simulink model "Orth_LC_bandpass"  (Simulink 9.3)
settings: Solver=VariableStepAuto  StartTime=0.0  StopTime=1  RelTol=1e-3
InitFcn:
  | Test_LibVishia_Ctrl.TestOrthOsc_init();
  | TstepHw=0.000001;
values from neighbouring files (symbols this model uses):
  Tstep = 0.000050    (= 5e-05)    [TestOrthOsc_init.m]    (also in Test_PIDctrl_init.m = 0.0001)
libraries: powerlib x12, libVishia_Ctrl x4, libVishia_Conv x2, libVishia_CtrlSfn x1, simulink x1

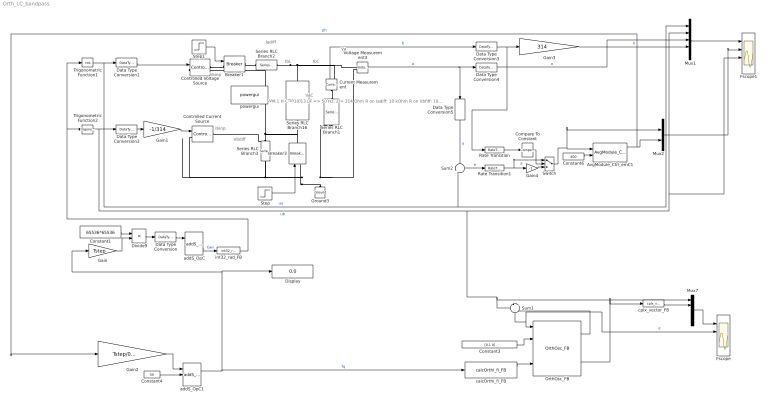
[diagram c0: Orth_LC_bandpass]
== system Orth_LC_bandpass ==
  note: L = 1 H C = 10.13 µF => 50 Hz, Z = 314 Ohm R on Iadiff: 10 kOhm R on Vbfiff: 10 Ohm => k ~ 0.03
  note: VaC
  note: Vainp
  note: Ibinp
  note: Vbdiff
  note: Iadiff
  note: IbC
  note: Va
  note: IbL
  note: VaL
  AvgModule_Ctrl_emC1 : libVishia_CtrlSfn/AvgModule_Ctrl_emC  SystemSampleTime=-1
  Breaker1 : powerlib/Elements/Breaker  InitialState=0  SwitchingTimes="[1/60  5/60]"  External=on  BreakerResistance=0.01  SnubberResistance=1e6  SnubberCapacitance=inf  Measurements=None  MoreParameters=on  NoBreakLoop=off
  Breaker3 : powerlib/Elements/Breaker  InitialState=0  SwitchingTimes="[1/60  5/60]"  External=on  BreakerResistance=0.01  SnubberResistance=1e6  SnubberCapacitance=inf  Measurements=None  MoreParameters=on  NoBreakLoop=off
  Compare To Constant : simulink/Logic and Bit Operations/Compare To Constant  relop=>=  const=0  OutDataTypeStr=boolean
  Constant1 : Constant  Value=65536*65536  OutDataTypeStr=single
  Constant3 : Constant  Value=[0.1 0]  OutDataTypeStr=single
  Constant4 : Constant  Value=50  OutDataTypeStr=single
  Constant6 : Constant  Value=400  OutDataTypeStr=single
  Controlled Current Source : powerlib/Electrical Sources/Controlled Current Source  Initialize=on  Source_Type=AC  Amplitude=0  Phase=0  Frequency=0  Measurements=None
  Controlled Voltage Source : powerlib/Electrical Sources/Controlled Voltage Source  Initialize=on  Source_Type=AC  Amplitude=0  Phase=0  Frequency=0  Measurements=None
  Current Measurement : powerlib/Measurements/Current Measurement  PhasorSimulation=off  OutputType=Complex  PSBequivalent=0
  Data Type Conversion : DataTypeConversion  OutDataTypeStr=int32
  Data Type Conversion1 : DataTypeConversion  OutDataTypeStr=double
  Data Type Conversion2 : DataTypeConversion  OutDataTypeStr=double
  Data Type Conversion3 : DataTypeConversion  OutDataTypeStr=single
  Data Type Conversion4 : DataTypeConversion  OutDataTypeStr=single
  Data Type Conversion5 : DataTypeConversion  OutDataTypeStr=single
  Display : Display
  Divide9 : Product  Inputs=**
  Fscope : Scope  NumInputPorts=4
  Fscope1 : Scope  NumInputPorts=4
  Gain : Gain  Gain=Tstep
  Gain1 : Gain  Gain=-1/314
  Gain2 : Gain  Gain=Tstep/0.1
  Gain3 : Gain  Gain=314
  Gain4 : Gain  Gain=-1
  Ground3 : powerlib/Elements/Ground  LConnTagsString=a
  Mux1 : Mux  Inputs=5
  Mux2 : Mux  Inputs=2
  Mux7 : Mux  Inputs=5
  OrthOsc_FB : libVishia_Ctrl/OrthOsc_FB
  Rate Transition : RateTransition  OutPortSampleTime=Tstep
  Rate Transition1 : RateTransition  OutPortSampleTime=Tstep
  Series RLC Branch1 : powerlib/Elements/Series RLC Branch  LConnTagsString=__new0  RConnTagsString=__new0  BranchType=C  Resistance=0  Inductance=0.001  SetiL0=off  InitialCurrent=0  Capacitance=10.13e-6  Setx0=off  InitialVoltage=0  Measurements=None
  Series RLC Branch16 : powerlib/Elements/Series RLC Branch  LConnTagsString=__new0  RConnTagsString=__new0  BranchType=L  Resistance=0  Inductance=1  SetiL0=off  InitialCurrent=0  Capacitance=100e-12  Setx0=off  InitialVoltage=0  Measurements=None
  Series RLC Branch2 : powerlib/Elements/Series RLC Branch  LConnTagsString=__new0  RConnTagsString=__new0  BranchType=R  Resistance=10000  Inductance=0.1  SetiL0=off  InitialCurrent=0  Capacitance=100e-12  Setx0=off  InitialVoltage=0  Measurements=None
  Series RLC Branch3 : powerlib/Elements/Series RLC Branch  LConnTagsString=__new0  RConnTagsString=__new0  BranchType=R  Resistance=10  Inductance=0.1  SetiL0=off  InitialCurrent=0  Capacitance=100e-12  Setx0=off  InitialVoltage=0  Measurements=None
  Step : Step  Time=0.6  SampleTime=0
  Step1 : Step  Time=0.2  SampleTime=0
  Sum1 : Sum  Inputs=+|-
  Sum2 : Sum  Inputs=-|+
  Switch : Switch  Criteria=u2 > Threshold
  Trigonometric Function1 : Trigonometry  Operator=cos
  Trigonometric Function2 : Trigonometry
  Voltage Measurement3 : powerlib/Measurements/Voltage Measurement  PhasorSimulation=off  OutputType=Complex  PSBequivalent=0
  addS_OpC : libVishia_Ctrl/addS_OpC  init=0  Tstep=Tstep
  addS_OpC1 : libVishia_Ctrl/addS_OpC  init=50  Tstep=Tstep
  calcOrthi_fi_FB : libVishia_Ctrl/calcOrthi_fi_FB  Tstep=Tstep
  cplx_vector_FB : libVishia_Conv/cplx_vector_FB  SystemSampleTime=-1
  int32_rad_FB : libVishia_Conv/int32_rad_FB  SystemSampleTime=-1
  powergui : powerlib/powergui  Priority=1  SimulationMode=Discrete  SampleTime=TstepHw  frequency=60  Iterations=50  frequencyindice=0  Pbase=100e6  ErrMax=1e-4  UnitsV=kV  UnitsW=MW  buscounter=0  FunctionMessages=off  echomessages=off  EnableUseOfTLC=off  CurrentSourceSwitches=off  DisableSnubberDevices=off  DisableRonSwitches=off  DisableVfSwitches=off  DisplayEquations=off  AutomaticDiscreteSolvers=off  SolverType=Tustin/Backward Euler (TBE)  Interpol=off  ExternalGateDelay=off  methode=off  Ts=100  x0status=blocks  SPID=on  SwTol=0  HookPort=off  NonlinearTolerance=0  nMaxIteration=15  ContinueOnMaxIteration=off  RestoreLinks=warning  ResistiveCurrentMeasurement=off  Frange=[0:2:500]  Ylog=off  Xlog=on  ShowGrid=off  save=off  variable=ZData  structure=0  ZoomFFT=off  StartTime=0.0  cycles=1  DisplayStyle=1  fundamental=60  FreqAxis=off  MaxFrequency=1000  frequencyindicesteady=1  RmsSteady=1  display=off
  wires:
  Constant3/1 -> OrthOsc_FB/3
  calcOrthi_fi_FB/1 -> OrthOsc_FB/7
  addS_OpC1/1 -> Display/1, Gain/1, calcOrthi_fi_FB/1  "fq"
  Data Type Conversion/1 -> addS_OpC/1
  int32_rad_FB/1 -> Trigonometric Function1/1, Trigonometric Function2/1
  addS_OpC/2 -> int32_rad_FB/1  "Gwi"
  Divide9/1 -> Data Type Conversion/1
  Gain/1 -> Divide9/2
  Trigonometric Function2/1 -> Fscope1/3, Mux1/2, Mux7/1, Sum1/1, Data Type Conversion2/1  "ub"
  Constant1/1 -> Divide9/1
  Mux7/1 -> Fscope/1
  cplx_vector_FB/1 -> Mux7/2
  OrthOsc_FB/3 -> cplx_vector_FB/1
  OrthOsc_FB/1 -> Sum1/2
  Sum1/1 -> Fscope/2, OrthOsc_FB/1  "e"
  Current Measurement/1 -> Data Type Conversion3/1  "b"
  Voltage Measurement3/1 -> Data Type Conversion4/1, Data Type Conversion5/1  "a"
  Data Type Conversion1/1 -> Controlled Voltage Source/1
  Trigonometric Function1/1 -> Sum2/2, Mux1/1, Data Type Conversion1/1  "ua"
  Data Type Conversion2/1 -> Gain1/1
  Gain1/1 -> Controlled Current Source/1
  Gain3/1 -> Mux1/4  "b"
  Mux1/1 -> Fscope1/1
  Data Type Conversion3/1 -> Rate Transition/1, Gain3/1
  Data Type Conversion4/1 -> Mux1/3  "a"
  Compare To Constant/1 -> Switch/2
  Switch/1 -> Mux2/1, AvgModule_Ctrl_emC1/1
  Rate Transition1/1 -> Switch/1, Gain4/1  "a"
  Gain4/1 -> Switch/3
  Constant6/1 -> AvgModule_Ctrl_emC1/2
  Sum2/1 -> Rate Transition1/1  "e"
  AvgModule_Ctrl_emC1/1 -> Gain2/1, Mux2/2  "ph"
  Mux2/1 -> Fscope1/2
  Rate Transition/1 -> Compare To Constant/1
  Constant4/1 -> addS_OpC1/2
  Gain2/1 -> addS_OpC1/1
  Step/1 -> Breaker3/1
  Step1/1 -> Breaker1/1
  Data Type Conversion5/1 -> Sum2/1  "a"
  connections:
  Ground3/LConn1 -- Voltage Measurement3/LConn2 -- Series RLC Branch1/LConn1 -- Controlled Current Source/LConn1 -- Controlled Voltage Source/LConn1 -- Series RLC Branch3/LConn1 -- Breaker3/LConn1
  Series RLC Branch1/RConn1 -- Current Measurement/LConn1
  Series RLC Branch2/RConn1 -- Current Measurement/RConn1 -- Voltage Measurement3/LConn1 -- Series RLC Branch16/RConn1
  Controlled Current Source/RConn1 -- Series RLC Branch16/LConn1 -- Breaker3/RConn1 -- Series RLC Branch3/RConn1
  Breaker1/RConn1 -- Series RLC Branch2/LConn1
  Breaker1/LConn1 -- Controlled Voltage Source/RConn1
